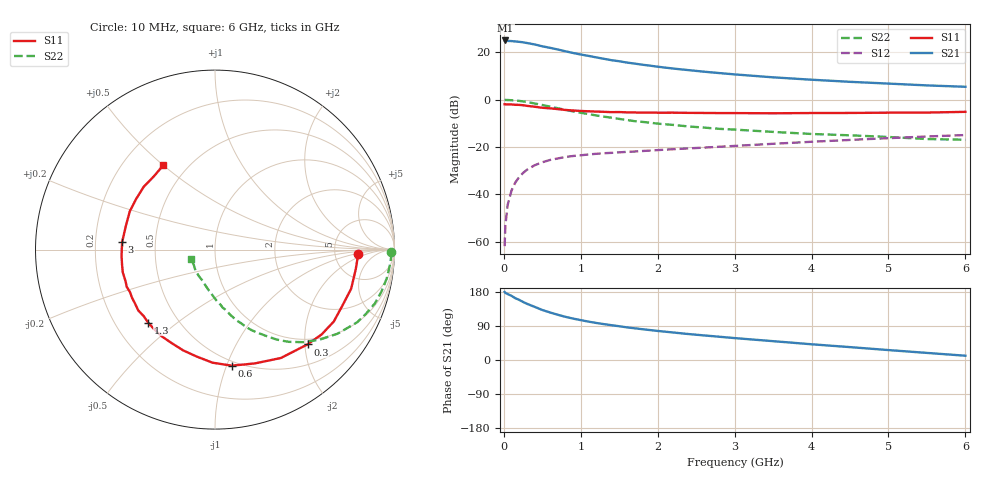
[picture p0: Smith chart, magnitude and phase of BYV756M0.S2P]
! SIEMENS Small Signal Semiconductors
! BFY420
! Si NPN RF SIEGET Grounded Emitter Transistor in MICRO-X
! VCE = 0.75 V  IC = 6 mA
! Common Emitter S-Parameters:  October  1996
# GHz  S  MA  R  50
!  f  S11  S21  S12  S22
! GHz  MAG  ANG  MAG  ANG  MAG  ANG  MAG  ANG
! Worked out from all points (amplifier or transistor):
!   36 points, 10 MHz to 6 GHz, reference 50 ohm
!   highest |S21| = 25.0 dB at 20 MHz (marker M1)
!   |S21| within 3 dB of that: start of sweep to 582.6 MHz
!   unconditionally stable (mu >= 1): 2.817 GHz to end of sweep
!   at 250 MHz: K = 0.13, MSG = 27.6 dB, |S12| = -31.0 dB
!   at 1.4 GHz: K = 0.62, MSG = 19.6 dB, |S12| = -22.5 dB
!   at 6 GHz: K = 1.16, MAG = 7.8 dB, |S12| = -15.0 dB
!   S11 on the Smith chart (normalised r, x): 10 MHz: 8.64, -1.25; 300 MHz: 0.89, -2.06; 600 MHz: 0.46, -1.04; 1.3 GHz: 0.34, -0.40; 3 GHz: 0.32, +0.04; 6 GHz: 0.37, +0.50
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0.01  0.7964 -1.9  17.72 179.7  0.0008 89.3  0.9812 -0.9
0.02  0.7954 -3.6  17.77 177.3  0.0022 84.8  0.9834 -1.8
0.05  0.7919 -7.9  17.35 174.0  0.006 87.7  0.9792 -4.7
0.1  0.7893 -16.0  17.24 169.3  0.012 82.1  0.9703 -9.5
0.15  0.7758 -23.4  16.93 163.0  0.0178 76.2  0.9564 -14.2
0.2  0.7737 -31.2  16.62 158.6  0.0232 73.9  0.9399 -18.6
0.25  0.7592 -38.5  16.22 153.2  0.0282 70.0  0.9143 -23.0
0.3  0.7379 -45.7  15.69 148.4  0.0329 66.9  0.8903 -27.0
0.4  0.7068 -58.7  14.64 140.3  0.041 60.8  0.8287 -34.4
0.5  0.6719 -70.7  13.37 132.0  0.0474 56.0  0.7687 -40.8
0.6  0.6535 -81.7  12.42 125.5  0.053 51.8  0.7109 -46.5
0.8  0.604 -99.9  10.49 114.0  0.0613 44.8  0.6074 -55.6
0.9  0.5891 -107.4  9.664 109.3  0.0643 43.1  0.5634 -59.0
1.1  0.567 -121.7  8.392 101.3  0.0694 39.9  0.494 -65.5
1.3  0.5515 -132.5  7.283 94.7  0.0737 37.8  0.4362 -70.4
1.7  0.5346 -149.8  5.761 83.7  0.08 35.3  0.3504 -78.8
2.2  0.5292 -166.2  4.532 72.6  0.0894 33.6  0.2918 -87.2
3  0.5189 175.3  3.41 57.8  0.105 31.9  0.2324 -98.0
3.5  0.5139 165.2  2.954 49.7  0.1165 30.2  0.2076 -104.7
4.5  0.5221 147.4  2.374 34.0  0.1406 24.9  0.1758 -119.0
5.5  0.532 129.6  1.995 18.7  0.1661 18.1  0.1467 -143.0
6  0.5512 121.6  1.865 11.3  0.1782 14.2  0.1418 -157.8
